(* Logix 5000 AddOnInstructionDefinition export AKD_Set_Motion_Task; software revision 20.04 *)

TYPE AKD_Status :   // All connections to the drive ethernet module are established and data is successfully transferring.
STRUCT
   Profile_In_Progress : BOOL;   // Profile Move In Progress
   Block_In_Execution : BOOL;   // Block In Execution
   On_Target_Position : BOOL;   // On Target Position (1=Current Position Equals Last Target Position)
   General_Fault : BOOL;   // General Fault
   Current_Direction : BOOL;   // Current Motor Direction (0=Reverse, 1=Forward)
   Home_Level : BOOL;   // Level of Home Input
   Reg_Level : BOOL;   // Level of Registration Input
   Enable : BOOL;   // State of Enable Output
   Fault_Input_Fault : BOOL;   // Fault Input Active
   Fwd_Limit : BOOL;   // Forward Input Active
   Rev_Limit : BOOL;   // Reverse Input Active
   Positive_Limit : BOOL;   // Positive Software Limit Exceeded
   Negative_Limit : BOOL;   // Negative Software Limit Exceeded
   FE_Fault : BOOL;   // Following Error Fault
   Block_Fault : BOOL;   // Block Execution Fault
   Load_Complete : BOOL;   // Command Message Successfully Loaded
END_STRUCT
END_TYPE

TYPE AKD_Control :   // Send Explicit Message
STRUCT
   Load_Data_Start_Profile : BOOL;   // Load Command Data / Start Profile Move
   Start_Block : BOOL;   // Execute Command block or block chain
   Incremental : BOOL;   // Incremental Position (0=Absolute, 1=Incremental)
   Direction : BOOL;   // Direction in Velocity Mode (0=Reverse, 1=Forward)
   Smooth_Stop : BOOL;   // Smooth / Controlled Stop w/ Deceleration
   Hard_Stop : BOOL;   // Hard / Immediate Stop
   Reg_Arm : BOOL;   // Arm the Registration Input
   Enable : BOOL;   // Enable Output
END_STRUCT
END_TYPE

TYPE AKD_Axis :   // Axis Data:
STRUCT
   Control : AKD_Control;   // Control bits to send to the drive
   Status : AKD_Status;   // Status bits received from the drive
   Input : AB:ETHERNET_MODULE_SINT_64Bytes:I:0;   // Data from the drive
   Output : AB:ETHERNET_MODULE_SINT_64Bytes:O:0;   // Data to the drive
   ResponseMsgType : SINT;   // Response type contained in latest IO response from drive. Used to check for errors
   CommandTimeout : INT;   // Time to allow for command response from drive. Dependent on scan rate and communicaiton rate
   PositionFeedback : DINT;   // Actual Position Value
   VelocityFeedback : DINT;   // Actual Velocity Value
END_STRUCT
END_TYPE

ADD_ON_INSTRUCTION AKD_Set_Motion_Task   (* revision 2.0, ExecutePrescan, ExecuteEnableInFalse *)
// Revision note:
// Changed MT.ACC, MT.DEC, MT.V, MT.P instances to 32 bit ( 4 byte ) instances. This allows MT.P to be set to negative values via the AOI.
VAR_OUTPUT
   DN : BOOL; {access Read Only, visible}   // Command Successful
   ER : BOOL; {access Read Only, visible}   // Error
END_VAR
VAR_IN_OUT
   Axis : AKD_Axis; {required}
END_VAR
VAR_INPUT
   MT_NUM : DINT; {required}   // Motion Task Number
   MT_ACC : DINT; {required}   // Motion Task Target Acc
   MT_DEC : DINT; {required}   // Motion Task Target DEC
   MT_V : DINT; {required}   // Motion Task Target Vel
   MT_P : DINT; {required}   // Motion Task Target Position
   MT_CNTL : DINT; {required}   // Motion Task Control Word
   MT_MTNEXT : DINT; {required}   // Following Motion Task Number
   MT_TNEXT : DINT; {required}   // Time Delay before following Motion Task is started
END_VAR
VAR
   Command_Timeout : TIMER := (PRE := 5000);   // Timeout Timer
   Command_Message_Type : SINT;   // Command Message Type
   Command_Axis_Number : SINT;   // Command Axis Number
   Step : SINT;
   Command_Bytes : SINT[8];
   OS_LoadStart : BOOL;
   Temp_Bytes : SINT[2];   // Temporary Bytes to Split into Command Bytes
   First_Scan_Bit : BOOL; {access None}
   MT_NUM_INSTANCE : DINT; {access None}
   MT_INSTANCE : DINT; {access None}
   MT_CMD_DATA : DINT; {access None}
END_VAR

ROUTINE EnableInFalse   (* ladder *)
// EnableIn_False
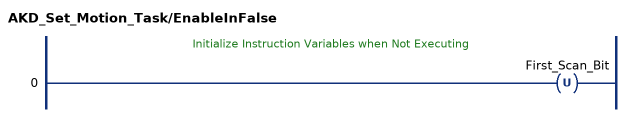
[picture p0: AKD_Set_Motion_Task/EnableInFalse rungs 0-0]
   // Initialize Instruction Variables when Not Executing
   0: OTU(First_Scan_Bit);
END_ROUTINE

ROUTINE Logic   (* ladder *)
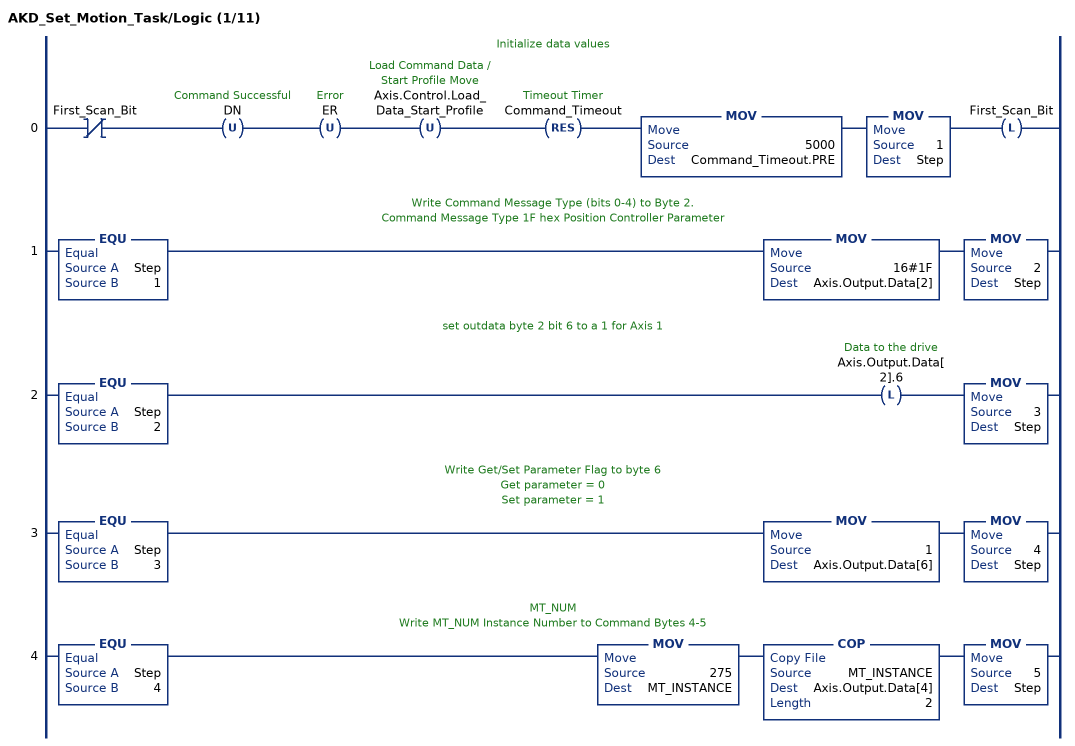
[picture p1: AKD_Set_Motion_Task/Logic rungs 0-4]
   // Initialize data values
   0: XIO(First_Scan_Bit)OTU(DN)OTU(ER)OTU(Axis.Control.Load_Data_Start_Profile)RES(Command_Timeout)MOV(5000,Command_Timeout.PRE)MOV(1,Step)OTL(First_Scan_Bit);
   // Write Command Message Type (bits 0-4) to Byte 2.
   // Command Message Type 1F hex Position Controller Parameter
   1: EQU(Step,1)MOV(16#1F,Axis.Output.Data[2])MOV(2,Step);
   // set outdata byte 2 bit 6 to a 1 for Axis 1
   2: EQU(Step,2)OTL(Axis.Output.Data[2].6)MOV(3,Step);
   // Write Get/Set Parameter Flag to byte 6
   // Get parameter = 0
   // Set parameter = 1
   3: EQU(Step,3)MOV(1,Axis.Output.Data[6])MOV(4,Step);
   // MT_NUM
   // Write MT_NUM Instance Number to Command Bytes 4-5
   4: EQU(Step,4)MOV(275,MT_INSTANCE)COP(MT_INSTANCE,Axis.Output.Data[4],2)MOV(5,Step);
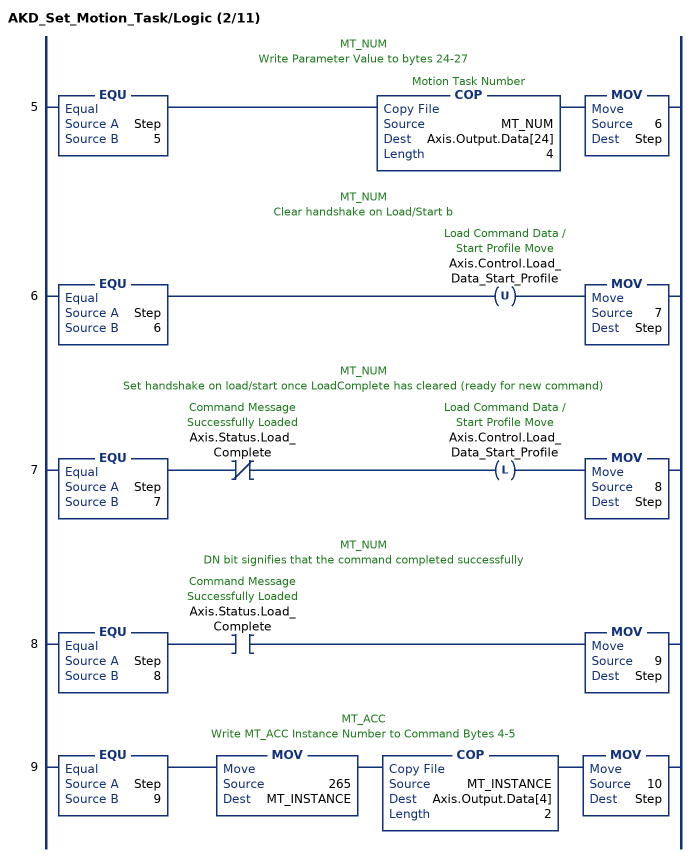
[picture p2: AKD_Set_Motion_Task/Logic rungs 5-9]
   // MT_NUM
   // Write Parameter Value to bytes 24-27
   5: EQU(Step,5)COP(MT_NUM,Axis.Output.Data[24],4)MOV(6,Step);
   // MT_NUM
   // Clear handshake on Load/Start b
   6: EQU(Step,6)OTU(Axis.Control.Load_Data_Start_Profile)MOV(7,Step);
   // MT_NUM
   // Set handshake on load/start once LoadComplete has cleared (ready for new command)
   7: EQU(Step,7)XIO(Axis.Status.Load_Complete)OTL(Axis.Control.Load_Data_Start_Profile)MOV(8,Step);
   // MT_NUM
   // DN bit signifies that the command completed successfully
   8: EQU(Step,8)XIC(Axis.Status.Load_Complete)MOV(9,Step);
   // MT_ACC
   // Write MT_ACC Instance Number to Command Bytes 4-5
   9: EQU(Step,9)MOV(265,MT_INSTANCE)COP(MT_INSTANCE,Axis.Output.Data[4],2)MOV(10,Step);
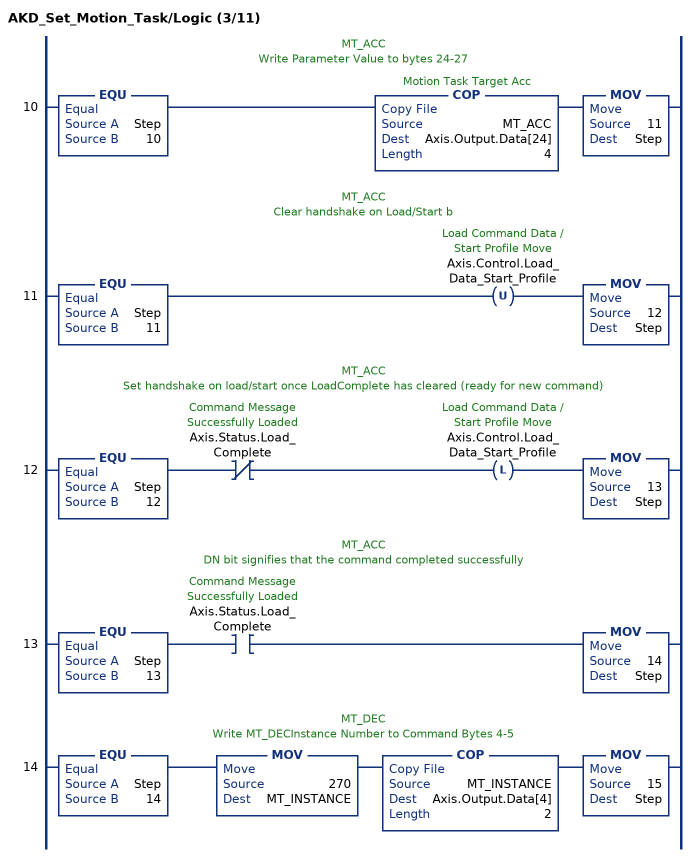
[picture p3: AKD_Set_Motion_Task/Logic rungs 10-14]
   // MT_ACC
   // Write Parameter Value to bytes 24-27
   10: EQU(Step,10)COP(MT_ACC,Axis.Output.Data[24],4)MOV(11,Step);
   // MT_ACC
   // Clear handshake on Load/Start b
   11: EQU(Step,11)OTU(Axis.Control.Load_Data_Start_Profile)MOV(12,Step);
   // MT_ACC
   // Set handshake on load/start once LoadComplete has cleared (ready for new command)
   12: EQU(Step,12)XIO(Axis.Status.Load_Complete)OTL(Axis.Control.Load_Data_Start_Profile)MOV(13,Step);
   // MT_ACC
   // DN bit signifies that the command completed successfully
   13: EQU(Step,13)XIC(Axis.Status.Load_Complete)MOV(14,Step);
   // MT_DEC
   // Write MT_DECInstance Number to Command Bytes 4-5
   14: EQU(Step,14)MOV(270,MT_INSTANCE)COP(MT_INSTANCE,Axis.Output.Data[4],2)MOV(15,Step);
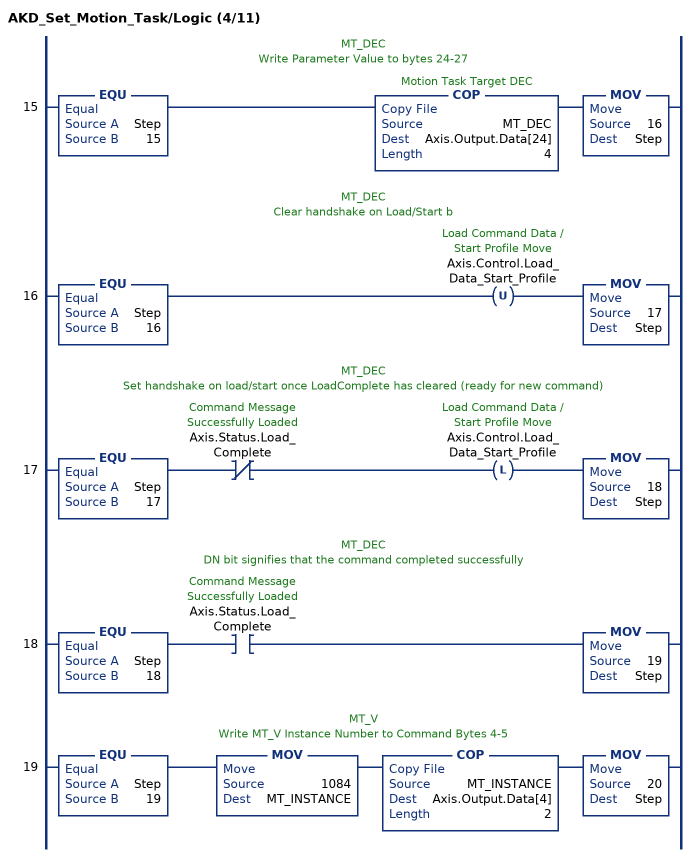
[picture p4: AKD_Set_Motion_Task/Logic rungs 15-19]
   // MT_DEC
   // Write Parameter Value to bytes 24-27
   15: EQU(Step,15)COP(MT_DEC,Axis.Output.Data[24],4)MOV(16,Step);
   // MT_DEC
   // Clear handshake on Load/Start b
   16: EQU(Step,16)OTU(Axis.Control.Load_Data_Start_Profile)MOV(17,Step);
   // MT_DEC
   // Set handshake on load/start once LoadComplete has cleared (ready for new command)
   17: EQU(Step,17)XIO(Axis.Status.Load_Complete)OTL(Axis.Control.Load_Data_Start_Profile)MOV(18,Step);
   // MT_DEC
   // DN bit signifies that the command completed successfully
   18: EQU(Step,18)XIC(Axis.Status.Load_Complete)MOV(19,Step);
   // MT_V
   // Write MT_V Instance Number to Command Bytes 4-5
   19: EQU(Step,19)MOV(1084,MT_INSTANCE)COP(MT_INSTANCE,Axis.Output.Data[4],2)MOV(20,Step);
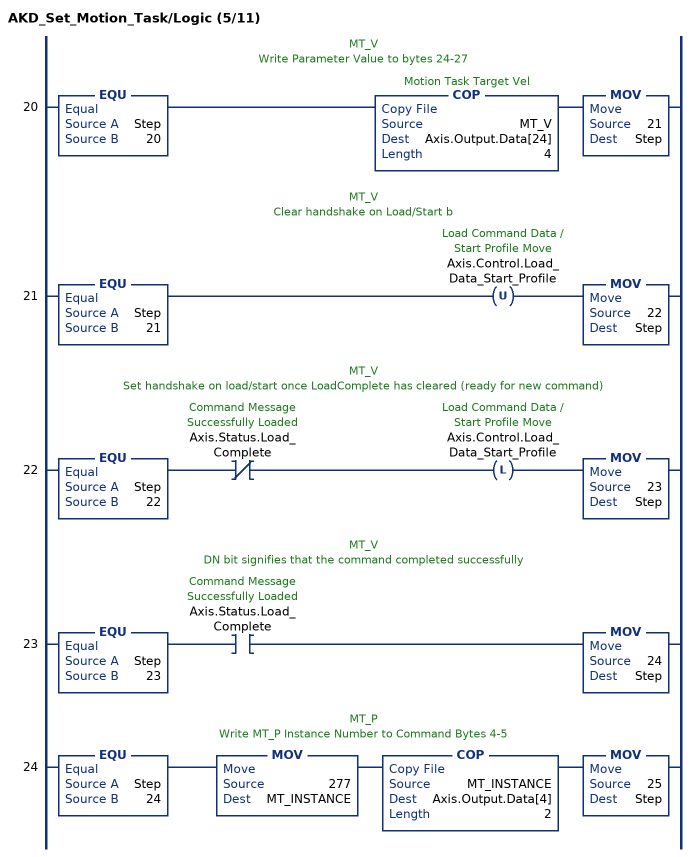
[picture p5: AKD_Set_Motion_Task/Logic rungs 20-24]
   // MT_V
   // Write Parameter Value to bytes 24-27
   20: EQU(Step,20)COP(MT_V,Axis.Output.Data[24],4)MOV(21,Step);
   // MT_V
   // Clear handshake on Load/Start b
   21: EQU(Step,21)OTU(Axis.Control.Load_Data_Start_Profile)MOV(22,Step);
   // MT_V
   // Set handshake on load/start once LoadComplete has cleared (ready for new command)
   22: EQU(Step,22)XIO(Axis.Status.Load_Complete)OTL(Axis.Control.Load_Data_Start_Profile)MOV(23,Step);
   // MT_V
   // DN bit signifies that the command completed successfully
   23: EQU(Step,23)XIC(Axis.Status.Load_Complete)MOV(24,Step);
   // MT_P
   // Write MT_P Instance Number to Command Bytes 4-5
   24: EQU(Step,24)MOV(277,MT_INSTANCE)COP(MT_INSTANCE,Axis.Output.Data[4],2)MOV(25,Step);
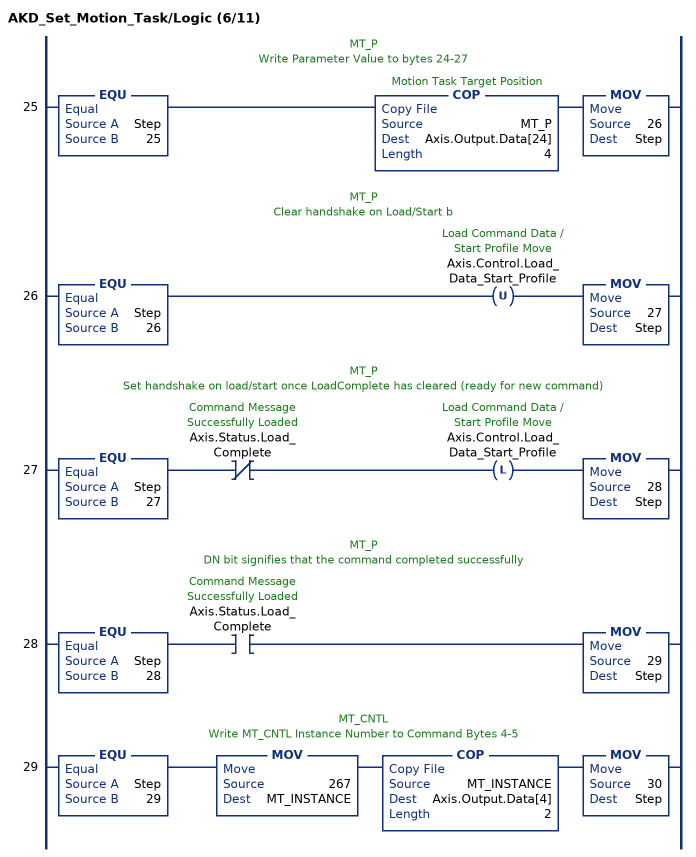
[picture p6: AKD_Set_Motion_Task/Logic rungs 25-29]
   // MT_P
   // Write Parameter Value to bytes 24-27
   25: EQU(Step,25)COP(MT_P,Axis.Output.Data[24],4)MOV(26,Step);
   // MT_P
   // Clear handshake on Load/Start b
   26: EQU(Step,26)OTU(Axis.Control.Load_Data_Start_Profile)MOV(27,Step);
   // MT_P
   // Set handshake on load/start once LoadComplete has cleared (ready for new command)
   27: EQU(Step,27)XIO(Axis.Status.Load_Complete)OTL(Axis.Control.Load_Data_Start_Profile)MOV(28,Step);
   // MT_P
   // DN bit signifies that the command completed successfully
   28: EQU(Step,28)XIC(Axis.Status.Load_Complete)MOV(29,Step);
   // MT_CNTL
   // Write MT_CNTL Instance Number to Command Bytes 4-5
   29: EQU(Step,29)MOV(267,MT_INSTANCE)COP(MT_INSTANCE,Axis.Output.Data[4],2)MOV(30,Step);
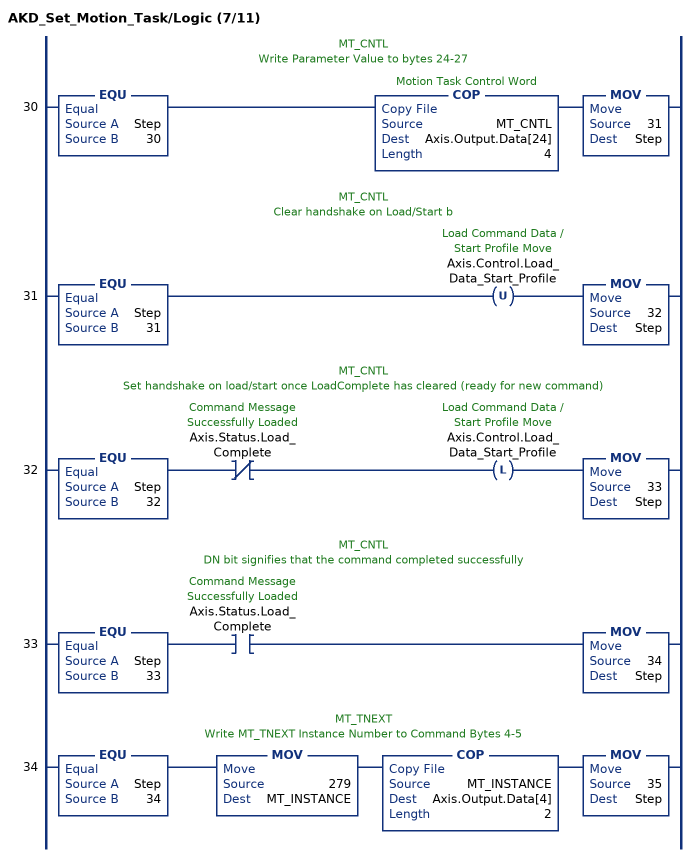
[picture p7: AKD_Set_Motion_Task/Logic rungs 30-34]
   // MT_CNTL
   // Write Parameter Value to bytes 24-27
   30: EQU(Step,30)COP(MT_CNTL,Axis.Output.Data[24],4)MOV(31,Step);
   // MT_CNTL
   // Clear handshake on Load/Start b
   31: EQU(Step,31)OTU(Axis.Control.Load_Data_Start_Profile)MOV(32,Step);
   // MT_CNTL
   // Set handshake on load/start once LoadComplete has cleared (ready for new command)
   32: EQU(Step,32)XIO(Axis.Status.Load_Complete)OTL(Axis.Control.Load_Data_Start_Profile)MOV(33,Step);
   // MT_CNTL
   // DN bit signifies that the command completed successfully
   33: EQU(Step,33)XIC(Axis.Status.Load_Complete)MOV(34,Step);
   // MT_TNEXT
   // Write MT_TNEXT Instance Number to Command Bytes 4-5
   34: EQU(Step,34)MOV(279,MT_INSTANCE)COP(MT_INSTANCE,Axis.Output.Data[4],2)MOV(35,Step);
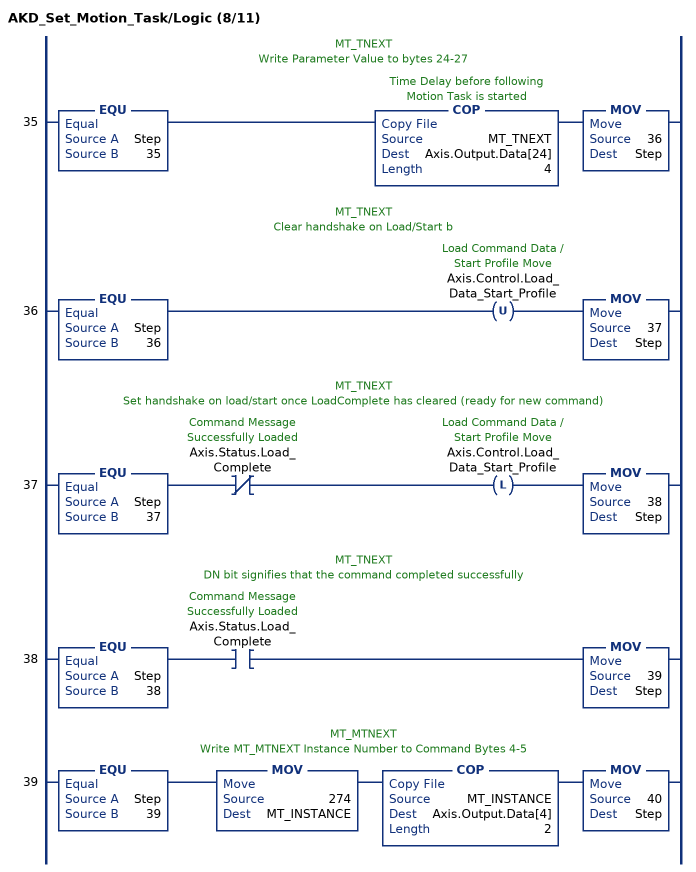
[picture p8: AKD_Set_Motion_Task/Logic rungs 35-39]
   // MT_TNEXT
   // Write Parameter Value to bytes 24-27
   35: EQU(Step,35)COP(MT_TNEXT,Axis.Output.Data[24],4)MOV(36,Step);
   // MT_TNEXT
   // Clear handshake on Load/Start b
   36: EQU(Step,36)OTU(Axis.Control.Load_Data_Start_Profile)MOV(37,Step);
   // MT_TNEXT
   // Set handshake on load/start once LoadComplete has cleared (ready for new command)
   37: EQU(Step,37)XIO(Axis.Status.Load_Complete)OTL(Axis.Control.Load_Data_Start_Profile)MOV(38,Step);
   // MT_TNEXT
   // DN bit signifies that the command completed successfully
   38: EQU(Step,38)XIC(Axis.Status.Load_Complete)MOV(39,Step);
   // MT_MTNEXT
   // Write MT_MTNEXT Instance Number to Command Bytes 4-5
   39: EQU(Step,39)MOV(274,MT_INSTANCE)COP(MT_INSTANCE,Axis.Output.Data[4],2)MOV(40,Step);
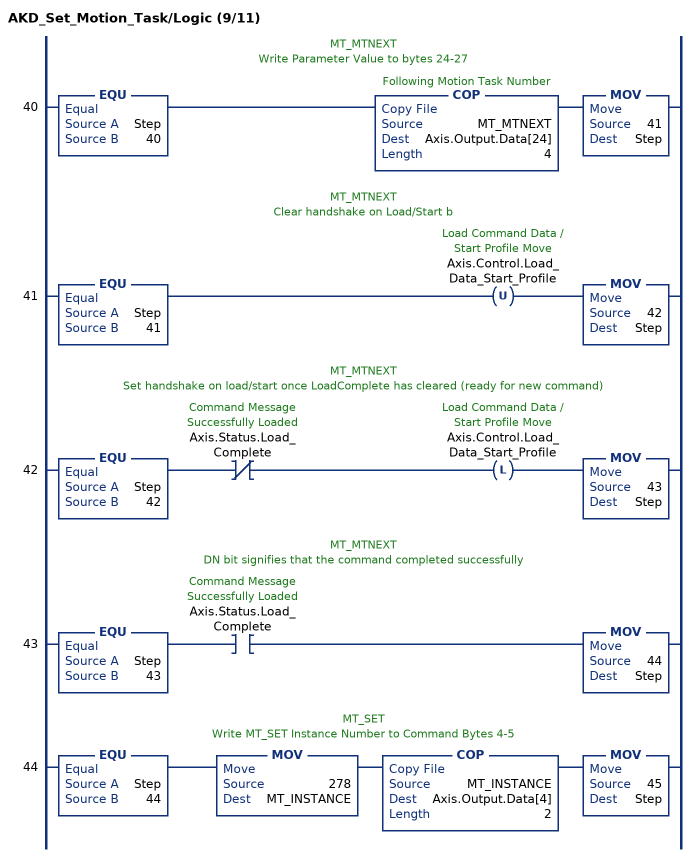
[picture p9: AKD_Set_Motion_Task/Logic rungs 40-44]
   // MT_MTNEXT
   // Write Parameter Value to bytes 24-27
   40: EQU(Step,40)COP(MT_MTNEXT,Axis.Output.Data[24],4)MOV(41,Step);
   // MT_MTNEXT
   // Clear handshake on Load/Start b
   41: EQU(Step,41)OTU(Axis.Control.Load_Data_Start_Profile)MOV(42,Step);
   // MT_MTNEXT
   // Set handshake on load/start once LoadComplete has cleared (ready for new command)
   42: EQU(Step,42)XIO(Axis.Status.Load_Complete)OTL(Axis.Control.Load_Data_Start_Profile)MOV(43,Step);
   // MT_MTNEXT
   // DN bit signifies that the command completed successfully
   43: EQU(Step,43)XIC(Axis.Status.Load_Complete)MOV(44,Step);
   // MT_SET
   // Write MT_SET Instance Number to Command Bytes 4-5
   44: EQU(Step,44)MOV(278,MT_INSTANCE)COP(MT_INSTANCE,Axis.Output.Data[4],2)MOV(45,Step);
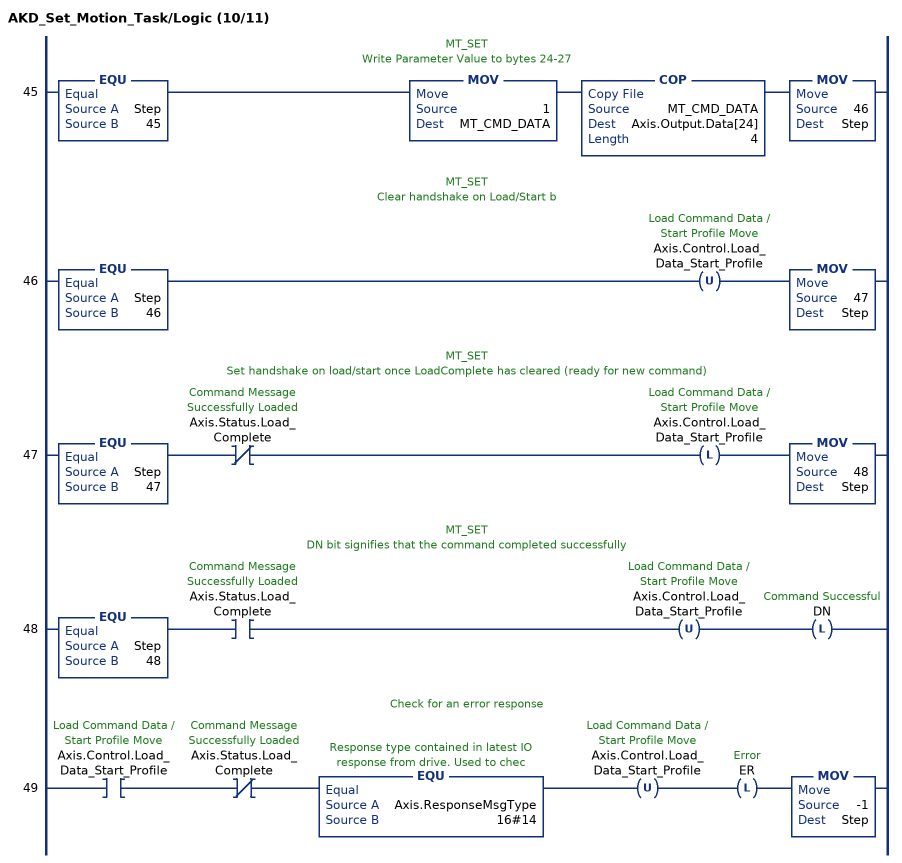
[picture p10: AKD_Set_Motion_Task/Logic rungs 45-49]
   // MT_SET
   // Write Parameter Value to bytes 24-27
   45: EQU(Step,45)MOV(1,MT_CMD_DATA)COP(MT_CMD_DATA,Axis.Output.Data[24],4)MOV(46,Step);
   // MT_SET
   // Clear handshake on Load/Start b
   46: EQU(Step,46)OTU(Axis.Control.Load_Data_Start_Profile)MOV(47,Step);
   // MT_SET
   // Set handshake on load/start once LoadComplete has cleared (ready for new command)
   47: EQU(Step,47)XIO(Axis.Status.Load_Complete)OTL(Axis.Control.Load_Data_Start_Profile)MOV(48,Step);
   // MT_SET
   // DN bit signifies that the command completed successfully
   48: EQU(Step,48)XIC(Axis.Status.Load_Complete)OTU(Axis.Control.Load_Data_Start_Profile)OTL(DN);
   // Check for an error response
   49: XIC(Axis.Control.Load_Data_Start_Profile)XIO(Axis.Status.Load_Complete)EQU(Axis.ResponseMsgType,16#14)OTU(Axis.Control.Load_Data_Start_Profile)OTL(ER)MOV(-1,Step);
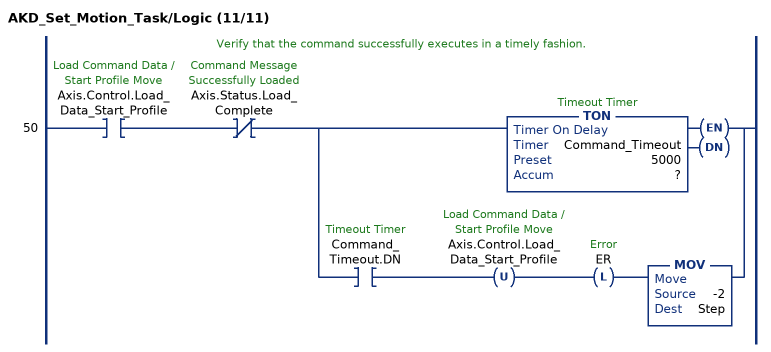
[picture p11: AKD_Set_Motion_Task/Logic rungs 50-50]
   // Verify that the command successfully executes in a timely fashion.
   50: XIC(Axis.Control.Load_Data_Start_Profile)XIO(Axis.Status.Load_Complete)[TON(Command_Timeout,?,?) ,XIC(Command_Timeout.DN) OTU(Axis.Control.Load_Data_Start_Profile) OTL(ER) MOV(-2,Step) ];
END_ROUTINE

ROUTINE Prescan   (* ladder *)
// Prescan
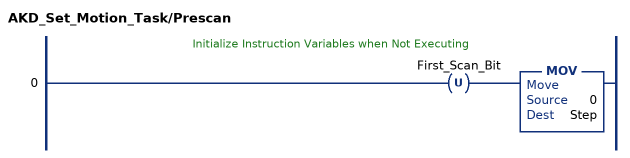
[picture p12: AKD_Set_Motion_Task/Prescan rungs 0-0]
   // Initialize Instruction Variables when Not Executing
   0: OTU(First_Scan_Bit)MOV(0,Step);
END_ROUTINE
END_ADD_ON_INSTRUCTION
